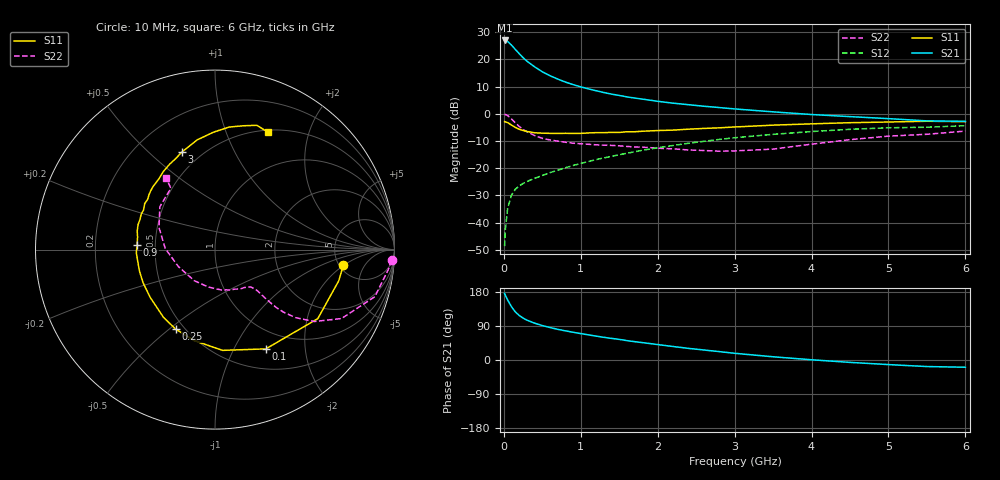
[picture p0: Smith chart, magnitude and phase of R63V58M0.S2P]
! SIEMENS Small Signal Semiconductors
! BFR193
! Si NPN RF Bipolar Junction Transistor in SOT23
! VCE = 3.5 V  IC = 8 mA
! Common Emitter S-Parameters:  May  1996
# GHz  S  MA  R  50
!  f  S11  S21  S12  S22
! GHz  MAG  ANG  MAG  ANG  MAG  ANG  MAG  ANG
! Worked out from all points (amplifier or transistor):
!   36 points, 10 MHz to 6 GHz, reference 50 ohm
!   highest |S21| = 27.0 dB at 10 MHz (marker M1)
!   |S21| within 3 dB of that: start of sweep to 139.7 MHz
!   unconditionally stable (mu >= 1): 790.2 MHz to 1.961 GHz
!   at 250 MHz: K = 0.57, MSG = 23.1 dB, |S12| = -25.6 dB
!   at 1.4 GHz: K = 1.04, MAG = 10.1 dB, |S12| = -15.6 dB
!   at 6 GHz: K = 0.95, MSG = 0.8 dB, |S12| = -4.4 dB
!   lowest NFmin = 1.25 dB at 450 MHz
!   S11 on the Smith chart (normalised r, x): 10 MHz: 5.40, -1.97; 100 MHz: 0.75, -1.35; 250 MHz: 0.45, -0.53; 900 MHz: 0.39, +0.03; 3 GHz: 0.39, +0.64; 6 GHz: 0.52, +1.42
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0.01  0.72 -7.0  22.29 175.6  0.0037 85.7  0.9851 -3.4
0.02  0.7112 -14.1  22.13 170.8  0.0076 85.7  0.9711 -6.7
0.05  0.6899 -33.9  21.33 158.0  0.0185 75.5  0.9285 -16.4
0.1  0.6214 -62.9  18.29 140.4  0.0321 63.4  0.8026 -28.6
0.15  0.563 -85.7  15.19 126.8  0.0412 57.4  0.6833 -35.9
0.2  0.52 -102.9  12.77 117.5  0.0472 54.1  0.5871 -40.2
0.25  0.4944 -116.3  10.75 110.6  0.0526 52.6  0.5167 -42.4
0.3  0.4742 -127.2  9.28 105.2  0.0571 52.9  0.4684 -43.4
0.4  0.4483 -143.8  7.301 97.2  0.0652 54.1  0.3984 -44.0
0.5  0.4413 -155.0  5.927 90.9  0.0737 56.1  0.3545 -44.1
0.6  0.4376 -164.0  5.008 85.7  0.083 57.3  0.3313 -44.1
0.7  0.4355 -171.7  4.354 81.0  0.0922 58.6  0.3151 -44.6
0.9  0.4351 176.4  3.446 73.2  0.1123 60.4  0.2883 -46.2
1.1  0.4455 166.6  2.873 66.3  0.1331 61.2  0.2755 -49.6
1.3  0.4504 158.0  2.462 59.9  0.1548 61.1  0.2654 -53.2
1.6  0.4682 146.8  2.047 51.1  0.1885 59.9  0.2517 -61.0
2.2  0.502 128.9  1.57 35.6  0.2621 55.2  0.2272 -81.5
3  0.5732 109.0  1.23 17.7  0.3635 45.0  0.2082 -123.5
3.5  0.6194 99.2  1.087 8.5  0.4196 37.4  0.2249 -155.0
4.5  0.687 83.5  0.888 -6.3  0.5192 22.0  0.3353 158.5
5.5  0.7306 71.4  0.742 -17.3  0.5672 6.1  0.4208 125.8
6  0.7177 65.7  0.727 -19.1  0.605 1.3  0.482 124.2
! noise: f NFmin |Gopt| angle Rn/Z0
0.45  1.25  0.23  133  0.12
0.9  1.3  0.35  156  0.11
1.8  2  0.55  -155  0.13
